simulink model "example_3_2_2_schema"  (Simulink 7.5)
settings: Solver=ode45  StartTime=0.0  StopTime=400  FixedStep=1e-3  RelTol=1e-3
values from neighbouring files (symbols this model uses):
  A = [0 0;1 0]    [example_3_2_2_podklad.m]
  B = [7.14;0]    [example_3_2_2_podklad.m]
  C = [0 1]    [example_3_2_2_podklad.m]
  D = 0    [example_3_2_2_podklad.m]
  Kreg = lqgreg(Kalmf,K)    [example_3_2_1_podklad.m]    (also in example_3_2_2_podklad.m = lqg(sys,QXU,QWV,QXI))
undefined symbols (not defined in the file or in its folder): K_r, Kalmf

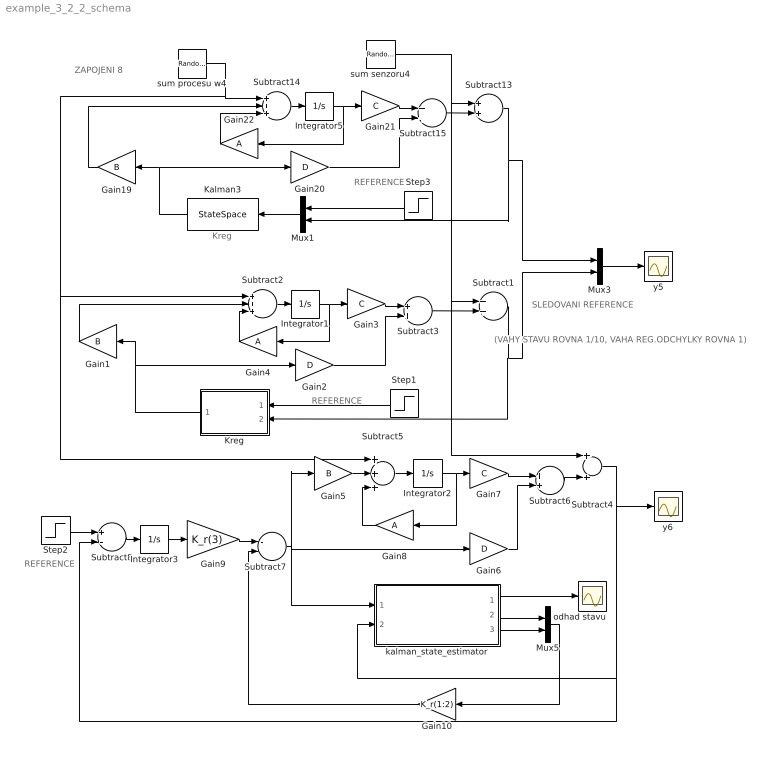
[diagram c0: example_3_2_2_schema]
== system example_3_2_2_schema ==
  note: Kreg
  note: SLEDOVANI REFERENCE
  note: (VAHY STAVU ROVNA 1/10, VAHA REG.ODCHYLKY ROVNA 1)
  note: ZAPOJENI 8
  note: REFERENCE
  note: REFERENCE
  note: REFERENCE
  Gain1 : Gain  Gain=B  Multiplication=Matrix(K*u)  ParameterDataType=sfix(16)  ParameterScaling=2^0  OutDataType=sfix(16)  OutScaling=2^0
  Gain10 : Gain  Gain=K_r(1:2)  Multiplication=Matrix(K*u)  ParameterDataType=sfix(16)  ParameterScaling=2^0  OutDataType=sfix(16)  OutScaling=2^0
  Gain19 : Gain  Gain=B  Multiplication=Matrix(K*u)  ParameterDataType=sfix(16)  ParameterScaling=2^0  OutDataType=sfix(16)  OutScaling=2^0
  Gain2 : Gain  Gain=D  Multiplication=Matrix(K*u)  ParameterDataType=sfix(16)  ParameterScaling=2^0  OutDataType=sfix(16)  OutScaling=2^0
  Gain20 : Gain  Gain=D  Multiplication=Matrix(K*u)  ParameterDataType=sfix(16)  ParameterScaling=2^0  OutDataType=sfix(16)  OutScaling=2^0
  Gain21 : Gain  Gain=C  Multiplication=Matrix(K*u)  ParameterDataType=sfix(16)  ParameterScaling=2^0  OutDataType=sfix(16)  OutScaling=2^0
  Gain22 : Gain  Gain=A  Multiplication=Matrix(K*u)  ParameterDataType=sfix(16)  ParameterScaling=2^0  OutDataType=sfix(16)  OutScaling=2^0
  Gain3 : Gain  Gain=C  Multiplication=Matrix(K*u)  ParameterDataType=sfix(16)  ParameterScaling=2^0  OutDataType=sfix(16)  OutScaling=2^0
  Gain4 : Gain  Gain=A  Multiplication=Matrix(K*u)  ParameterDataType=sfix(16)  ParameterScaling=2^0  OutDataType=sfix(16)  OutScaling=2^0
  Gain5 : Gain  Gain=B  Multiplication=Matrix(K*u)  ParameterDataType=sfix(16)  ParameterScaling=2^0  OutDataType=sfix(16)  OutScaling=2^0
  Gain6 : Gain  Gain=D  Multiplication=Matrix(K*u)  ParameterDataType=sfix(16)  ParameterScaling=2^0  OutDataType=sfix(16)  OutScaling=2^0
  Gain7 : Gain  Gain=C  Multiplication=Matrix(K*u)  ParameterDataType=sfix(16)  ParameterScaling=2^0  OutDataType=sfix(16)  OutScaling=2^0
  Gain8 : Gain  Gain=A  Multiplication=Matrix(K*u)  ParameterDataType=sfix(16)  ParameterScaling=2^0  OutDataType=sfix(16)  OutScaling=2^0
  Gain9 : Gain  Gain=K_r(3)  ParameterDataType=sfix(16)  ParameterScaling=2^0  OutDataType=sfix(16)  OutScaling=2^0
  Integrator{1..3,5} (4 alike) : Integrator
  Kalman3 : StateSpace  A=Kreg.a  B=Kreg.b  C=Kreg.c  D=Kreg.d
  Kreg : Subsystem
  Mux1 : Mux  Inputs=2
  Mux3 : Mux  Inputs=2
  Mux5 : Mux  Inputs=2
  Step1 : Step  Time=50  Before=400  After=0  SampleTime=0
  Step2 : Step  Time=50  Before=400  After=0  SampleTime=0
  Step3 : Step  Time=50  Before=400  After=0  SampleTime=0
  Subtract{1,3..4,6,13,15} (6 alike) : Sum  OutDataType=sfix(16)  OutScaling=2^-10
  Subtract14 : Sum  Inputs=+++  OutDataType=sfix(16)  OutScaling=2^-10
  Subtract2 : Sum  Inputs=+++  OutDataType=sfix(16)  OutScaling=2^-10
  Subtract5 : Sum  Inputs=+++  OutDataType=sfix(16)  OutScaling=2^-10
  Subtract7 : Sum  Inputs=--  OutDataType=sfix(16)  OutScaling=2^-10
  Subtract8 : Sum  Inputs=+-  OutDataType=sfix(16)  OutScaling=2^-10
  kalman_state_estimator : Subsystem
  odhad stavu : Scope
  sum procesu w4 : RandomNumber  Variance=0.02  SampleTime=0
  sum senzoru4 : RandomNumber  Variance=0.02  SampleTime=0
  y5 : Scope
  y6 : Scope
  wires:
  Integrator5/1 -> Gain22/1, Gain21/1
  Subtract14/1 -> Integrator5/1
  Subtract15/1 -> Subtract13/2
  Gain21/1 -> Subtract15/1
  Gain20/1 -> Subtract15/2
  Gain22/1 -> Subtract14/3
  Gain19/1 -> Subtract14/2
  Mux1/1 -> Kalman3/1
  Subtract13/1 -> Mux1/2, Mux3/1
  sum procesu w4/1 -> Subtract14/1, Subtract2/1, Subtract5/1
  Kalman3/1 -> Gain19/1, Gain20/1
  Step3/1 -> Mux1/1
  Integrator1/1 -> Gain3/1, Gain4/1
  Subtract2/1 -> Integrator1/1
  Subtract3/1 -> Subtract1/2
  Gain3/1 -> Subtract3/1
  Gain2/1 -> Subtract3/2
  Gain4/1 -> Subtract2/3
  Gain1/1 -> Subtract2/2
  Subtract1/1 -> Kreg/2(y), Mux3/2
  Kreg/1(u) -> Gain2/1, Gain1/1
  Integrator2/1 -> Gain8/1, Gain7/1
  Subtract5/1 -> Integrator2/1
  Subtract6/1 -> Subtract4/2
  Gain7/1 -> Subtract6/1
  Gain6/1 -> Subtract6/2
  Gain8/1 -> Subtract5/3
  Gain5/1 -> Subtract5/2
  Integrator3/1 -> Gain9/1
  Subtract8/1 -> Integrator3/1
  Gain9/1 -> Subtract7/1
  Subtract7/1 -> kalman_state_estimator/1(u), Gain5/1, Gain6/1
  Subtract4/1 -> kalman_state_estimator/2(y), Subtract8/2, y6/1
  kalman_state_estimator/2(x1_kalman) -> Mux5/1
  kalman_state_estimator/3(x2_kalman) -> Mux5/2
  Mux5/1 -> Gain10/1
  Gain10/1 -> Subtract7/2
  Step1/1 -> Kreg/1(ref)
  Step2/1 -> Subtract8/1
  Mux3/1 -> y5/1
  kalman_state_estimator/1(y_kalman) -> odhad stavu/1
  sum senzoru4/1 -> Subtract13/1, Subtract1/1, Subtract4/1

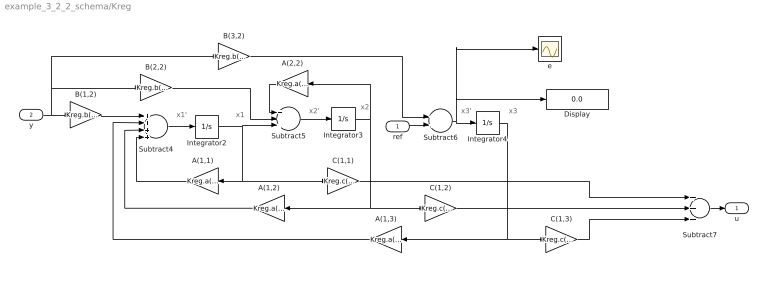
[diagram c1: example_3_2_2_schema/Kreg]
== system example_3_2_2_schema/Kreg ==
  note: x1'
  note: x1
  note: x2'
  note: x2
  note: x3
  note: x3'
  ref : Inport  OutDataType=fixdt(1, 16)  OutScaling=2^0
  y : Inport  Port=2  OutDataType=fixdt(1, 16)  OutScaling=2^0
  A(1,1) : Gain  Gain=Kreg.a(1,1)  ParameterDataType=sfix(16)  ParameterScaling=2^0  OutDataType=sfix(16)  OutScaling=2^0
  A(1,2) : Gain  Gain=Kreg.a(1,2)  ParameterDataType=sfix(16)  ParameterScaling=2^0  OutDataType=sfix(16)  OutScaling=2^0
  A(1,3) : Gain  Gain=Kreg.a(1,3)  ParameterDataType=sfix(16)  ParameterScaling=2^0  OutDataType=sfix(16)  OutScaling=2^0
  A(2,2) : Gain  Gain=Kreg.a(2,2)  ParameterDataType=sfix(16)  ParameterScaling=2^0  OutDataType=sfix(16)  OutScaling=2^0
  B(1,2) : Gain  Gain=Kreg.b(1,2)  ParameterDataType=sfix(16)  ParameterScaling=2^0  OutDataType=sfix(16)  OutScaling=2^0
  B(2,2) : Gain  Gain=Kreg.b(2,2)  ParameterDataType=sfix(16)  ParameterScaling=2^0  OutDataType=sfix(16)  OutScaling=2^0
  B(3,2) : Gain  Gain=Kreg.b(3,2)  ParameterDataType=sfix(16)  ParameterScaling=2^0  OutDataType=sfix(16)  OutScaling=2^0
  C(1,1) : Gain  Gain=Kreg.c(1,1)  ParameterDataType=sfix(16)  ParameterScaling=2^0  OutDataType=sfix(16)  OutScaling=2^0
  C(1,2) : Gain  Gain=Kreg.c(1,2)  ParameterDataType=sfix(16)  ParameterScaling=2^0  OutDataType=sfix(16)  OutScaling=2^0
  C(1,3) : Gain  Gain=Kreg.c(1,3)  ParameterDataType=sfix(16)  ParameterScaling=2^0  OutDataType=sfix(16)  OutScaling=2^0
  Display : Display
  Integrator2 : Integrator
  Integrator3 : Integrator
  Integrator4 : Integrator
  Subtract4 : Sum  Inputs=++++  OutDataType=sfix(16)  OutScaling=2^-10
  Subtract5 : Sum  Inputs=+++  OutDataType=sfix(16)  OutScaling=2^-10
  Subtract6 : Sum  OutDataType=sfix(16)  OutScaling=2^-10
  Subtract7 : Sum  Inputs=+++  OutDataType=sfix(16)  OutScaling=2^-10
  e : Scope
  u : Outport  OutDataType=fixdt(1, 16)  OutScaling=2^0
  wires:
  Subtract4/1 -> Integrator2/1
  Integrator2/1 -> Subtract5/3, A(1,1)/1, C(1,1)/1
  Subtract5/1 -> Integrator3/1
  Integrator3/1 -> A(2,2)/1, A(1,2)/1, C(1,2)/1
  Integrator4/1 -> A(1,3)/1, C(1,3)/1
  A(1,1)/1 -> Subtract4/4
  A(1,2)/1 -> Subtract4/3
  A(1,3)/1 -> Subtract4/2
  A(2,2)/1 -> Subtract5/1
  B(1,2)/1 -> Subtract4/1
  y/1 -> B(1,2)/1, B(2,2)/1, B(3,2)/1
  B(2,2)/1 -> Subtract5/2
  Subtract6/1 -> Integrator4/1, e/1, Display/1
  B(3,2)/1 -> Subtract6/1
  ref/1 -> Subtract6/2
  C(1,1)/1 -> Subtract7/1
  C(1,2)/1 -> Subtract7/2
  C(1,3)/1 -> Subtract7/3
  Subtract7/1 -> u/1

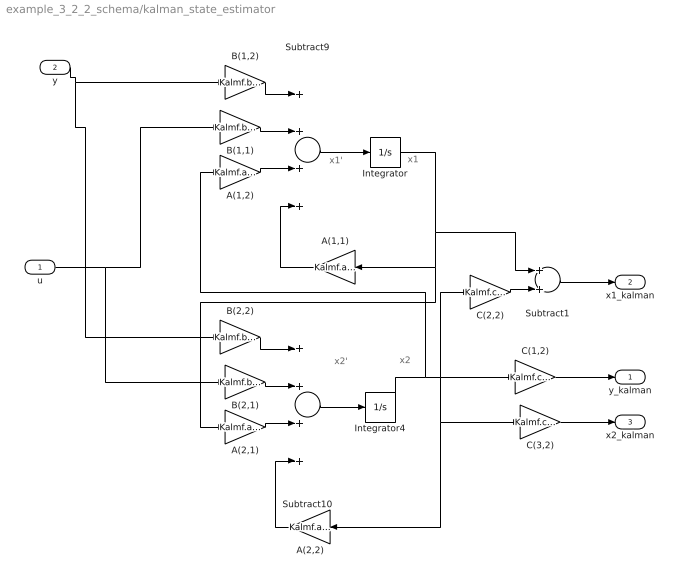
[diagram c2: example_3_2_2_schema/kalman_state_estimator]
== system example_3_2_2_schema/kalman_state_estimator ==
  note: x2
  note: x2'
  note: x1
  note: x1'
  u : Inport
  y : Inport  Port=2
  A(1,1) : Gain  Gain=Kalmf.a(1,1)  ParameterDataType=sfix(16)  ParameterScaling=2^0  OutDataType=sfix(16)  OutScaling=2^0
  A(1,2) : Gain  Gain=Kalmf.a(1,2)  ParameterDataType=sfix(16)  ParameterScaling=2^0  OutDataType=sfix(16)  OutScaling=2^0
  A(2,1) : Gain  Gain=Kalmf.a(2,1)  ParameterDataType=sfix(16)  ParameterScaling=2^0  OutDataType=sfix(16)  OutScaling=2^0
  A(2,2) : Gain  Gain=Kalmf.a(2,2)  ParameterDataType=sfix(16)  ParameterScaling=2^0  OutDataType=sfix(16)  OutScaling=2^0
  B(1,1) : Gain  Gain=Kalmf.b(1,1)  ParameterDataType=sfix(16)  ParameterScaling=2^0  OutDataType=sfix(16)  OutScaling=2^0
  B(1,2) : Gain  Gain=Kalmf.b(1,2)  ParameterDataType=sfix(16)  ParameterScaling=2^0  OutDataType=sfix(16)  OutScaling=2^0
  B(2,1) : Gain  Gain=Kalmf.b(2,1)  ParameterDataType=sfix(16)  ParameterScaling=2^0  OutDataType=sfix(16)  OutScaling=2^0
  B(2,2) : Gain  Gain=Kalmf.b(2,2)  ParameterDataType=sfix(16)  ParameterScaling=2^0  OutDataType=sfix(16)  OutScaling=2^0
  C(1,2) : Gain  Gain=Kalmf.c(1,2)  ParameterDataType=sfix(16)  ParameterScaling=2^0  OutDataType=sfix(16)  OutScaling=2^0
  C(2,2) : Gain  Gain=Kalmf.c(2,2)  ParameterDataType=sfix(16)  ParameterScaling=2^0  OutDataType=sfix(16)  OutScaling=2^0
  C(3,2) : Gain  Gain=Kalmf.c(3,2)  ParameterDataType=sfix(16)  ParameterScaling=2^0  OutDataType=sfix(16)  OutScaling=2^0
  Integrator : Integrator
  Integrator4 : Integrator
  Subtract1 : Sum  OutDataType=sfix(16)  OutScaling=2^-10
  Subtract10 : Sum  Inputs=++++  OutDataType=sfix(16)  OutScaling=2^-10
  Subtract9 : Sum  Inputs=++++  OutDataType=sfix(16)  OutScaling=2^-10
  y_kalman : Outport
  x1_kalman : Outport  Port=2
  x2_kalman : Outport  Port=3
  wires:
  C(3,2)/1 -> x2_kalman/1
  Subtract1/1 -> x1_kalman/1
  C(2,2)/1 -> Subtract1/2
  C(1,2)/1 -> y_kalman/1
  B(2,2)/1 -> Subtract10/1
  B(2,1)/1 -> Subtract10/2
  Integrator4/1 -> A(2,2)/1, C(3,2)/1, C(2,2)/1, C(1,2)/1, A(1,2)/1
  A(2,1)/1 -> Subtract10/3
  Subtract10/1 -> Integrator4/1
  y/1 -> B(1,2)/1, B(2,2)/1
  B(1,2)/1 -> Subtract9/1
  u/1 -> B(1,1)/1, B(2,1)/1
  B(1,1)/1 -> Subtract9/2
  A(1,1)/1 -> Subtract9/4
  Integrator/1 -> A(1,1)/1, A(2,1)/1, Subtract1/1
  A(1,2)/1 -> Subtract9/3
  Subtract9/1 -> Integrator/1
  A(2,2)/1 -> Subtract10/4
